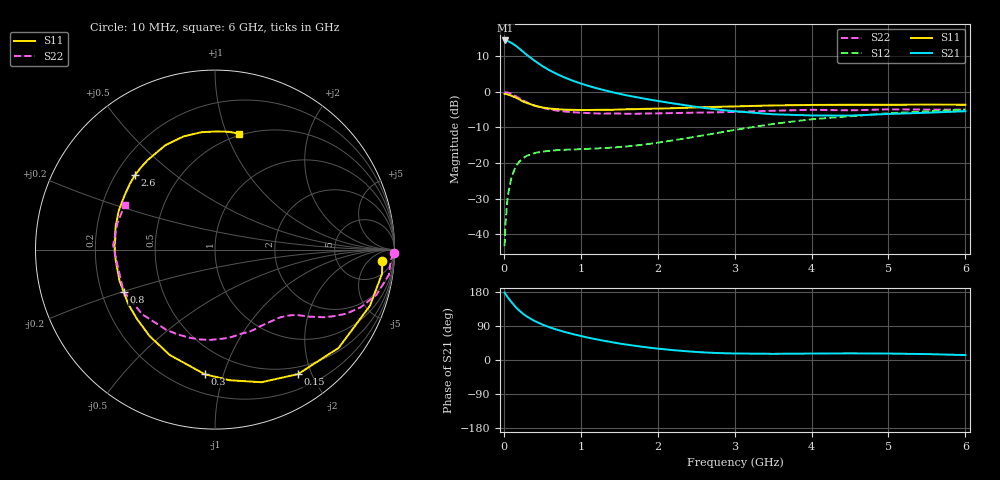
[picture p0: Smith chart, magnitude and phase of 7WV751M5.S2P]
! Infineon Technologies  Discrete & RF Semiconductors
! BFS17W
! Si NPN RF Bipolar Junction Transistor in SOT323
! VCE = 0.75 V  IC = 1.5 mA
! Common Emitter S-Parameters:  August  1999
# GHz  S  MA  R  50
!  f  S11  S21  S12  S22
! GHz  MAG  ANG  MAG  ANG  MAG  ANG  MAG  ANG
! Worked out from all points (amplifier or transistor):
!   36 points, 10 MHz to 6 GHz, reference 50 ohm
!   highest |S21| = 14.4 dB at 20 MHz (marker M1)
!   |S21| within 3 dB of that: start of sweep to 241.2 MHz
!   unconditionally stable (mu >= 1): 817 MHz to end of sweep
!   at 250 MHz: K = 0.34, MSG = 14.9 dB, |S12| = -18.6 dB
!   at 1.4 GHz: K = 1.42, MAG = 4.0 dB, |S12| = -15.7 dB
!   at 6 GHz: K = 1.14, MAG = -2.5 dB, |S12| = -5.0 dB
!   S11 on the Smith chart (normalised r, x): 10 MHz: 15, -15; 150 MHz: 0.40, -1.80; 300 MHz: 0.32, -0.87; 800 MHz: 0.29, -0.20; 2.6 GHz: 0.28, +0.37; 6 GHz: 0.48, +1.11
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0.01  0.9346 -3.9  5.265 177.9  0.0068 86.0  0.9982 -1.2
0.02  0.9402 -8.3  5.269 174.4  0.0134 85.0  0.9815 -3.3
0.05  0.9183 -19.9  5.179 165.6  0.034 78.7  0.9788 -8.3
0.1  0.8801 -38.5  4.861 152.7  0.0634 67.7  0.9343 -15.6
0.15  0.8337 -56.3  4.485 140.5  0.0875 58.9  0.873 -21.6
0.2  0.783 -70.7  4.067 130.6  0.1046 52.0  0.8143 -26.0
0.25  0.7323 -83.6  3.662 122.0  0.1172 45.8  0.7567 -29.4
0.3  0.6968 -94.7  3.298 114.8  0.1268 41.7  0.713 -31.9
0.4  0.6392 -113.2  2.733 102.8  0.1384 35.5  0.6414 -35.6
0.5  0.604 -127.1  2.306 93.7  0.1447 31.8  0.5957 -37.9
0.6  0.5816 -138.4  1.989 85.9  0.1487 29.7  0.5655 -40.2
0.8  0.561 -155.2  1.575 73.5  0.1537 28.0  0.5275 -45.5
1.1  0.5559 -173.1  1.212 58.7  0.1586 29.4  0.5029 -54.1
1.3  0.5596 177.3  1.06 50.7  0.1627 31.6  0.4951 -60.8
1.6  0.5692 166.1  0.891 40.5  0.1713 36.0  0.4915 -71.1
2.2  0.5889 147.9  0.688 26.0  0.2084 44.9  0.5034 -92.7
2.6  0.6092 137.0  0.595 20.0  0.2454 48.0  0.512 -107.3
3.5  0.6442 115.4  0.484 16.3  0.3543 45.8  0.5427 -138.4
4  0.6545 105.5  0.466 17.0  0.412 40.8  0.5597 -155.8
4.5  0.6585 96.5  0.464 17.5  0.454 35.3  0.55 -170.7
5.5  0.661 83.3  0.509 15.6  0.5322 24.9  0.5632 164.6
6  0.659 78.3  0.534 13.0  0.564 19.8  0.5607 153.8
